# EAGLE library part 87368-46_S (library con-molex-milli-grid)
RECEPTACAL
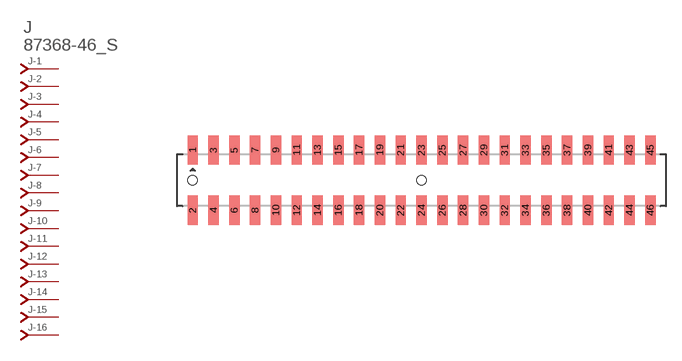
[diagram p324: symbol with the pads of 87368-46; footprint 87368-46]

Designator prefix J; gates -1=J-NV -2=J-N -3=J-N -4=J-N -5=J-N -6=J-N -7=J-N -8=J-N -9=J-N -10=J-N -11=J-N -12=J-N -13=J-N -14=J-N -15=J-N -16=J-N -17=J-N -18=J-N -19=J-N -20=J-N -21=J-N -22=J-N -23=J-N -24=J-N -25=J-N -26=J-N -27=J-N -28=J-N -29=J-N -30=J-N -31=J-N -32=J-N -33=J-N -34=J-N -35=J-N -36=J-N -37=J-N -38=J-N -39=J-N -40=J-N -41=J-N -42=J-N -43=J-N -44=J-N -45=J-N -46=J-N

## 87368-46_S  [87368-46]
1  -1:J  pas
2  -2:J  pas
3  -3:J  pas
4  -4:J  pas
5  -5:J  pas
6  -6:J  pas
7  -7:J  pas
8  -8:J  pas
9  -9:J  pas
10  -10:J  pas
11  -11:J  pas
12  -12:J  pas
13  -13:J  pas
14  -14:J  pas
15  -15:J  pas
16  -16:J  pas
17  -17:J  pas
18  -18:J  pas
19  -19:J  pas
20  -20:J  pas
21  -21:J  pas
22  -22:J  pas
23  -23:J  pas
24  -24:J  pas
25  -25:J  pas
26  -26:J  pas
27  -27:J  pas
28  -28:J  pas
29  -29:J  pas
30  -30:J  pas
31  -31:J  pas
32  -32:J  pas
33  -33:J  pas
34  -34:J  pas
35  -35:J  pas
36  -36:J  pas
37  -37:J  pas
38  -38:J  pas
39  -39:J  pas
40  -40:J  pas
41  -41:J  pas
42  -42:J  pas
43  -43:J  pas
44  -44:J  pas
45  -45:J  pas
46  -46:J  pas

## Footprint 87368-46 (pad centres in mm)
RECEPTACAL SMD Dual Row, Side Entry
smd 1 x 2.8: 1 -22,2.9; 2 -22,-2.9; 3 -20,2.9; 4 -20,-2.9; 5 -18,2.9; 6 -18,-2.9; 7 -16,2.9; 8 -16,-2.9; 9 -14,2.9; 10 -14,-2.9; 11 -12,2.9; 12 -12,-2.9; 13 -10,2.9; 14 -10,-2.9; 15 -8,2.9; 16 -8,-2.9; 17 -6,2.9; 18 -6,-2.9; 19 -4,2.9; 20 -4,-2.9; 21 -2,2.9; 22 -2,-2.9; 23 0,2.9; 24 0,-2.9; 25 2,2.9; 26 2,-2.9; 27 4,2.9; 28 4,-2.9; 29 6,2.9; 30 6,-2.9; 31 8,2.9; 32 8,-2.9; 33 10,2.9; 34 10,-2.9; 35 12,2.9; 36 12,-2.9; 37 14,2.9; 38 14,-2.9; 39 16,2.9; 40 16,-2.9; 41 18,2.9; 42 18,-2.9; 43 20,2.9; 44 20,-2.9; 45 22,2.9; 46 22,-2.9
hole 0.914 at -22,0
hole 0.914 at 0,0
